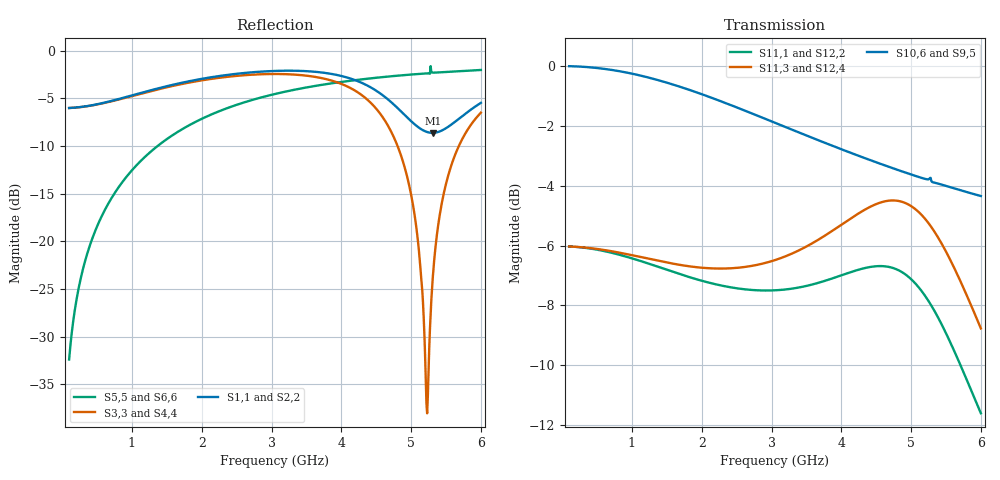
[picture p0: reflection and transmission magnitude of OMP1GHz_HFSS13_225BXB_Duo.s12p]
! Touchstone file from project OMP1GHz_HFSS13
! Exported from HFSS 13.0.2
! Variables:
!  PCB_bot = -0.459mm
!  PCB_t = 0.762mm
!  PCB_top = 0.303mm
!  PCB_x = 10mm
!  baseplate_x = 30.2mm
!  bot = -1.27mm
!  deem_x = 9.9mm
!  gap = 100um
!  heatsink_x = 10mm
!  heatsink_y = 40mm
!  lead_bot = 0.303mm
!  lead_ext_ref = 5.2mm
!  lead_w = 3.85mm
# GHZ S MA R 50.000000
! Terminal data exported
! Port[1] = Cdummy_a_T1
! Port[2] = Cdummy_b_T1
! Port[3] = Cinshin_a_T1
! Port[4] = Cinshin_b_T1
! Port[5] = Cpre_a_T1
! Port[6] = Cpre_b_T1
! Port[7] = iDrain_a_T1
! Port[8] = iDrain_b_T1
! Port[9] = in_a2_T1
! Port[10] = in_b2_T1
! Port[11] = out_a1_T1
! Port[12] = out_b1_T1
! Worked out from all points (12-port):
!   591 points, 100 MHz to 6 GHz, reference 50 ohm
!   strongest paths, dB at 100 MHz, 1.57 GHz, 3.05 GHz, 4.53 GHz, 6 GHz:
!     S10,6: 0.0, -0.6, -1.9, -3.2, -4.3
!     S9,5: 0.0, -0.6, -1.9, -3.2, -4.4
!     S11,3: -6.0, -6.6, -6.5, -4.6, -8.8
!     S12,4: -6.0, -6.6, -6.5, -4.6, -8.8
!     S11,1: -6.0, -6.9, -7.5, -6.7, -11.6
!     S12,2: -6.0, -6.9, -7.5, -6.7, -11.6
!   lowest |S11| = -8.6 dB at 5.31 GHz (marker M1), VSWR 2.18, Z = 23 - j1.12 ohm
!   |S11| at or under -10 dB: nowhere
